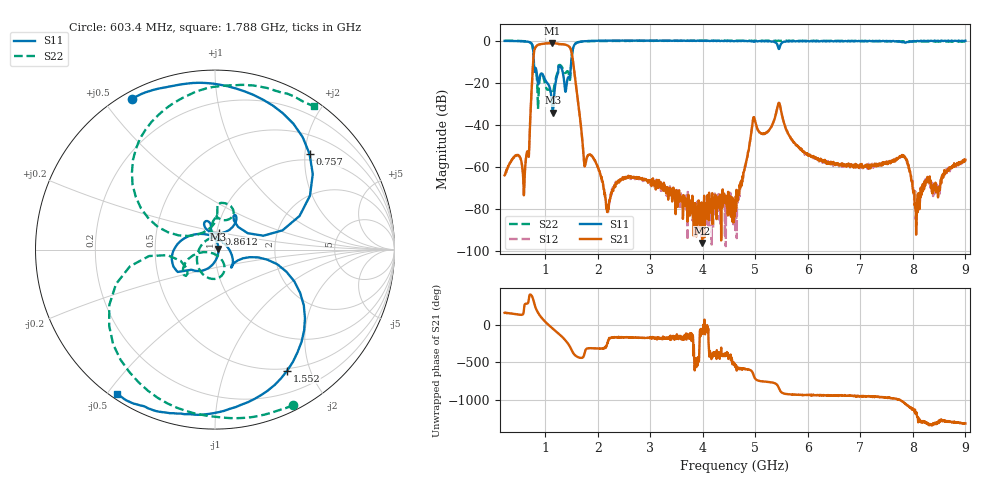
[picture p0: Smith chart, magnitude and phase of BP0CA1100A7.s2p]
!Agilent Technologies,E8358A,US41080443,A.07.50.56
!Agilent E8358A: A.07.50.56
!Date: Tuesday, April 11, 2017 15:47:19
!Correction: S11(Full 2 Port(1,2))
!S21(Full 2 Port(1,2))
!S12(Full 2 Port(1,2))
!S22(Full 2 Port(1,2))
!S2P File: Measurements: S11, S21, S12, S22:
# Hz S  dB  R 50
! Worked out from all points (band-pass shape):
!   1601 points, 225 MHz to 9 GHz, reference 50 ohm
!   highest |S21| = -1.18 dB at 1.135 GHz (marker M1); lowest = -96.3 dB at 3.987 GHz (marker M2)
!   |S21| within 3 dB of the highest: 794.3 MHz to 1.486 GHz (691.8 MHz wide, 60.7 % of centre)
!   lowest |S11| = -34.2 dB at 1.141 GHz (marker M3), VSWR 1.04, Z = 52 + j0.301 ohm
!   |S11| at or under -10 dB: 782.4 MHz to 1.494 GHz (711.3 MHz wide, 62.5 % of centre)
!   |S22| runs from -32.6 to 0.1 dB; largest |S21 - S12| = 0.01
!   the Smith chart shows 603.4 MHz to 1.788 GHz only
!   S11 on the Smith chart (normalised r, x): 603.4 MHz: 0.03, +0.59; 757 MHz: 0.86, +2.10; 861.2 MHz: 1.02, +0.19; 1.552 GHz: 0.47, -1.66; 1.788 GHz: 0.02, -0.53
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2.25e8  -0.11 163.5  -64.10 159.2  -64.01 158.2  -0.01 -16.0
6.034219e8  -0.36 118.8  -67.20 -97.9  -66.48 -100.2  -0.25 -63.3
7.569844e8  -2.51 45.3  -15.08 3.0  -15.17 3.4  -2.77 -144.1
8.611875e8  -20.72 77.5  -1.97 160.3  -2.06 160.4  -32.58 -114.9
9.599062e8  -16.48 100.6  -1.44 68.8  -1.52 69.0  -17.07 -129.0
1.135406e9  -32.97 34.4  -1.18 -46.9  -1.26 -46.9  -25.34 77.0
1.140891e9  -34.23 8.6  -1.18 -50.3  -1.27 -50.2  -25.10 81.6
1.338328e9  -15.79 152.2  -1.70 -172.2  -1.79 -172.2  -13.63 62.4
1.437047e9  -17.39 -45.7  -2.48 105.9  -2.57 105.8  -14.91 86.9
1.552219e9  -2.10 -59.2  -14.69 -33.6  -14.76 -33.8  -1.99 116.3
1.689328e9  -0.40 -109.0  -43.19 -78.7  -43.33 -78.9  -0.48 70.1
1.788047e9  -0.24 -124.0  -56.03 43.9  -56.03 42.2  -0.27 55.4
2.182922e9  -0.00 -150.1  -80.43 120.6  -80.01 88.5  -0.11 24.9
3.153656e9  -0.04 -171.1  -70.02 176.6  -67.37 -175.0  -0.02 -8.0
3.987281e9  -0.09 178.2  -96.27 -91.7  -85.09 -167.9  -0.03 -24.0
4.6125e9  -0.13 170.6  -77.50 -158.3  -83.42 96.7  -0.04 -34.1
4.974469e9  -0.52 163.9  -36.46 36.3  -36.45 37.7  -0.04 -37.3
5.451609e9  -3.95 159.9  -29.66 -125.1  -29.64 -125.3  -0.00 -44.1
6.076828e9  -0.26 146.6  -55.19 149.3  -55.10 145.7  -0.09 -51.5
7.541156e9  -0.26 125.1  -57.68 110.8  -57.23 112.3  -0.21 -83.6
8.084109e9  -0.10 122.4  -75.73 -146.3  -73.29 -138.8  -0.43 -99.1
9e9  0.00 111.6  -56.71 130.6  -57.18 130.1  -0.49 -125.5
